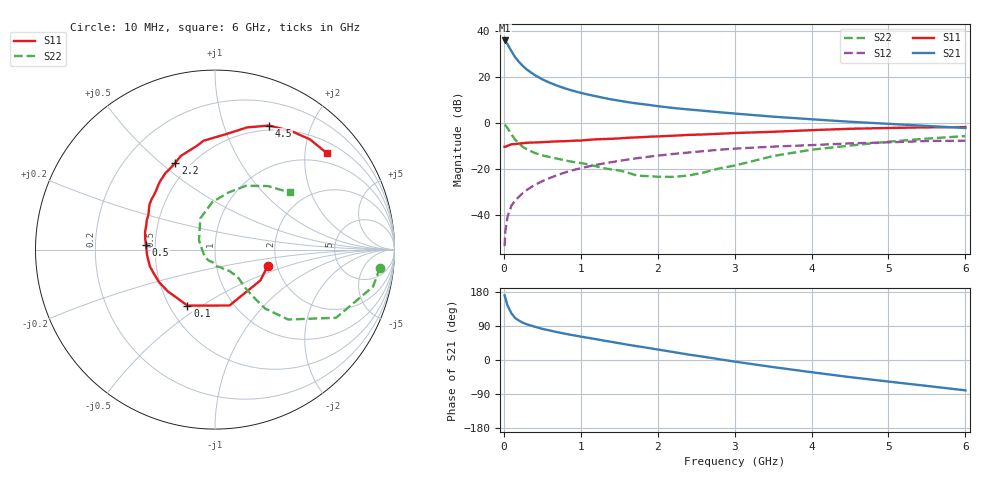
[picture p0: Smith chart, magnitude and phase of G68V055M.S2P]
! SIEMENS Small Signal Semiconductors
! BFG193
! Si NPN RF Bipolar Junction Transistor in SOT223
! VCE = 8 V  IC = 55 mA
! Common Emitter S-Parameters:  August  1996
# GHz  S  MA  R  50
!  f  S11  S21  S12  S22
! GHz  MAG  ANG  MAG  ANG  MAG  ANG  MAG  ANG
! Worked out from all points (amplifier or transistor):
!   36 points, 10 MHz to 6 GHz, reference 50 ohm
!   highest |S21| = 36.0 dB at 10 MHz (marker M1)
!   |S21| within 3 dB of that: start of sweep to 70.62 MHz
!   unconditionally stable (mu >= 1): 465.1 MHz to 2.395 GHz
!   at 250 MHz: K = 0.90, MSG = 27.5 dB, |S12| = -30.3 dB
!   at 1.4 GHz: K = 1.04, MAG = 12.4 dB, |S12| = -17.0 dB
!   at 6 GHz: K = 0.89, MSG = 2.8 dB, |S12| = -7.6 dB
!   S11 on the Smith chart (normalised r, x): 10 MHz: 1.79, -0.35; 100 MHz: 0.62, -0.44; 500 MHz: 0.44, +0.03; 2.2 GHz: 0.42, +0.56; 4.5 GHz: 0.45, +1.43; 6 GHz: 0.75, +2.49
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0.01  0.3072 -17.0  63.13 170.6  0.0021 86.8  0.9251 -6.2
0.02  0.3061 -34.0  60.81 163.3  0.0045 81.0  0.9042 -13.2
0.05  0.3218 -75.5  51.44 142.6  0.0095 72.1  0.774 -29.4
0.1  0.3475 -116.2  36.57 122.7  0.0162 66.7  0.5637 -43.7
0.15  0.3509 -138.4  26.89 110.4  0.021 65.5  0.4316 -49.6
0.2  0.3606 -149.8  21.24 103.5  0.0255 67.8  0.3567 -50.7
0.25  0.3667 -159.2  17.32 98.1  0.0305 67.6  0.3014 -51.4
0.3  0.3746 -165.5  14.66 94.1  0.0353 68.7  0.2705 -51.7
0.4  0.3798 -175.6  11.18 88.0  0.045 69.1  0.2249 -50.9
0.5  0.3855 175.9  8.982 82.2  0.0546 68.1  0.1981 -50.3
0.6  0.3938 171.2  7.546 77.7  0.0643 66.9  0.1825 -51.1
0.7  0.4019 165.8  6.491 73.3  0.0748 66.1  0.1682 -53.0
0.8  0.4057 160.9  5.681 69.2  0.0848 64.1  0.1539 -54.7
1.1  0.4323 148.4  4.169 58.4  0.114 59.1  0.1262 -64.3
1.3  0.4518 141.3  3.541 51.2  0.133 55.2  0.1045 -71.3
1.6  0.4792 131.2  2.889 40.7  0.1604 48.4  0.0853 -90.1
2.2  0.5323 114.5  2.142 21.1  0.2136 35.0  0.0679 -151.3
2.8  0.5869 99.9  1.731 2.1  0.2639 21.1  0.1032 149.8
3.5  0.6487 84.0  1.385 -18.7  0.3087 4.0  0.1926 115.1
4.5  0.7543 66.4  1.073 -45.2  0.3631 -15.9  0.3255 77.1
5.5  0.8107 49.2  0.87 -68.4  0.409 -39.2  0.4608 50.2
6  0.8225 40.8  0.784 -80.1  0.4153 -52.6  0.5234 37.5
